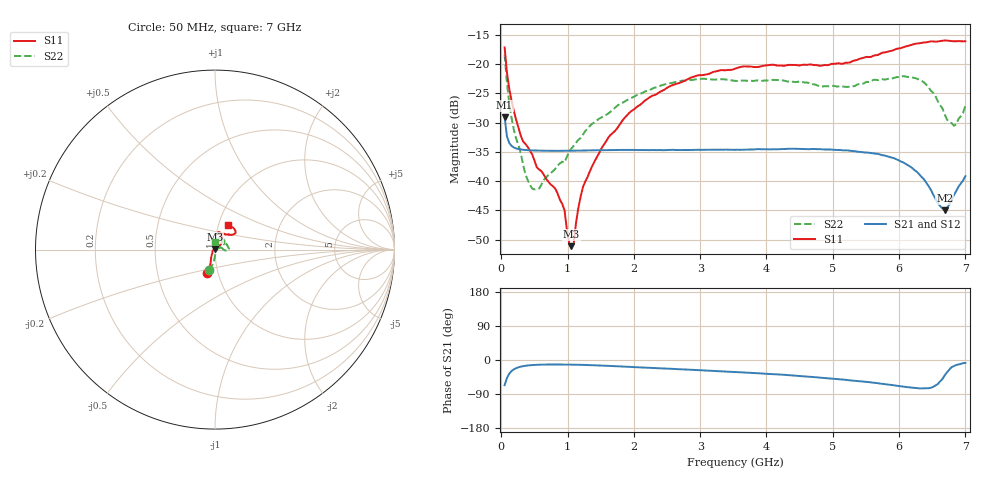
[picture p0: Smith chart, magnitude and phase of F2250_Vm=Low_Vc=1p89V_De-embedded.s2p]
! Integrated Device Technology
! Corporate Headquarters
! 6024 Silver Creek Valley Road
! San Jose, CA 95138  USA
! Phone:  1-408-284-8200
! Toll Free:  1-800-223-1366
! Webpage:  http://www.idt.com/
! Timing and RF Division
! 515 Groton Road, Suite 102
! Westford, MA 01886-6024
! Device:  F2250
! Description: Voltage Variable RF Attenuator
! Frequency:  50.0 -  6000.00 MHz
! Package:  3x3 mm Thin QFN Plastic Package: 16 pin
! Ports:  2 RF, 3 DC
!  Pin  1  = GND
!  Pin  2  = NC
!  Pin  3  = RF1  = Port 1
!  Pin  4  = NC
!  Pin  5  = GND
!  Pin  6  = GND
!  Pin  7  = GND
!  Pin  8  = GND
!  Pin  9  = NC
!  Pin 10  = RF2  = Port 2
!  Pin 11  = NC
!  Pin 12  = GND
!  Pin 13  = GND
!  Pin 14  = VCNTRL
!  Pin 15  = VDD
!  Pin 16  = VMODE
! Vcntrl:  1.890 Volts
! Vmode:  +0.000 Volts
! Vdd:  +3.30  Volts
! Current:  1.184 mA
! Data:  The device was measured on a the F2250 evaluation board which has
!  individual transmission lines to the RF pins.  Data was collected
!  using a calibrated network analyzer.  The evaluation board was
!  de-embedded using a TRL calibration technique.
!  The reference plane is the edge of the package pin.
! Misc:  SN 10
!  Action Tracker AT0258
! Date Measured:  2014-11-26
! Date:  2015-10-15  MJV
! Note:
!  Integrated Device Technology supplies this data as a sample of measured
!  data at the package pin for this product.  Your particular data for this
!  product may vary.
!  Data was taken at 25 degrees C.
!  Integrated Device Technology reserves the right to change this data at anytime.
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# GHz S dB R 50
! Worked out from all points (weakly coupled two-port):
!   201 points, 50 MHz to 7 GHz, reference 50 ohm
!   highest |S21| = -29.09 dB at 50 MHz (marker M1); lowest = -45.0 dB at 6.687 GHz (marker M2)
!   lowest |S11| = -51.1 dB at 1.058 GHz (marker M3), VSWR 1.01, Z = 49.9 + j0.238 ohm
!   |S11| at or under -10 dB: start of sweep to end of sweep
!   |S22| runs from -41.4 to -18.4 dB; largest |S21 - S12| = 6.1e-05
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0.05  -17.17 -108.5  -29.09 -66.4  -29.09 -66.4  -18.38 -105.0
0.08475  -21.44 -107.3  -32.33 -47.4  -32.33 -47.4  -23.18 -95.4
0.189  -28.01 -119.4  -34.26 -24.7  -34.26 -24.7  -31.20 -87.2
0.328  -33.21 -133.3  -34.65 -16.3  -34.65 -16.3  -37.13 -61.6
0.467  -35.45 -146.8  -34.76 -13.3  -34.75 -13.3  -41.28 -26.0
0.57125  -38.02 -159.9  -34.79 -12.4  -34.80 -12.4  -41.26 -8.3
0.91875  -43.88 157.9  -34.83 -11.9  -34.84 -11.9  -36.67 14.6
0.9535  -44.95 170.0  -34.83 -11.9  -34.83 -11.9  -36.80 20.0
1.023  -50.51 142.9  -34.83 -12.1  -34.83 -12.1  -34.97 21.6
1.05775  -51.10 120.9  -34.83 -12.2  -34.82 -12.2  -34.43 22.9
1.0925  -50.68 86.0  -34.81 -12.3  -34.81 -12.3  -33.97 22.0
1.162  -44.59 54.7  -34.80 -12.5  -34.80 -12.6  -32.97 19.9
1.2315  -41.02 43.3  -34.77 -12.9  -34.77 -12.9  -32.06 18.6
1.61375  -32.58 40.5  -34.71 -15.5  -34.71 -15.5  -28.44 26.7
2.37825  -24.87 47.1  -34.69 -21.8  -34.69 -21.7  -23.85 35.5
3.525  -20.82 72.4  -34.66 -31.6  -34.66 -31.7  -22.89 62.0
4.7065  -20.18 72.3  -34.51 -45.0  -34.51 -45.0  -23.48 64.5
5.85325  -17.83 40.4  -35.86 -65.2  -35.86 -65.3  -22.49 10.3
6.3745  -16.34 41.3  -39.68 -75.0  -39.69 -75.0  -23.14 -4.3
6.68725  -15.99 48.8  -44.99 -40.8  -44.99 -40.6  -28.58 15.9
6.82625  -16.14 53.6  -42.41 -15.9  -42.35 -15.9  -30.53 51.5
7  -16.13 63.2  -39.14 -7.8  -39.10 -8.0  -27.08 93.2
